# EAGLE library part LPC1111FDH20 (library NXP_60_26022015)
32-bit ARM Cortex-M0 microcontroller; up to 64 kB flash and 8 kB SRAM The LPC1110/11/12/13/14/15 are a ARM Cortex-M0 based, low-cost 32-bit MCU family, designed for 8/16-bit microcontroller applications, offering performance, low power, simple instruction set and memory addressing together with reduced code size compared to existing 8/16-bit architectures. The LPC1110/11/12/13/14/15 operate at CPU frequencies of up to 50 MHz. The peripheral complement of the LPC1110/11/12/13/14/15 includes up to 64 kB of flash memory, up to 8 kB of data memory, one Fast-mode Plus I 2 C-bus interface, one RS-485/EIA-485 UART, up to two SPI interfaces with SSP features, four general purpose counter/timers, a 10-bit ADC, and up to 42 general purpose I/O pins. Remark: The LPC111x series consists of the LPC1100 series (parts LPC111x/101/201/301), LPC1100L series (parts LPC111x/002/102/202/302), and the LPC1100XL series (parts LPC111x/103/203/303/323/333). The LPC1100L and LPC1100XL series include the power profiles, a windowed watchdog timer, and a configurable open-drain mode. AAL Eindhoven MK
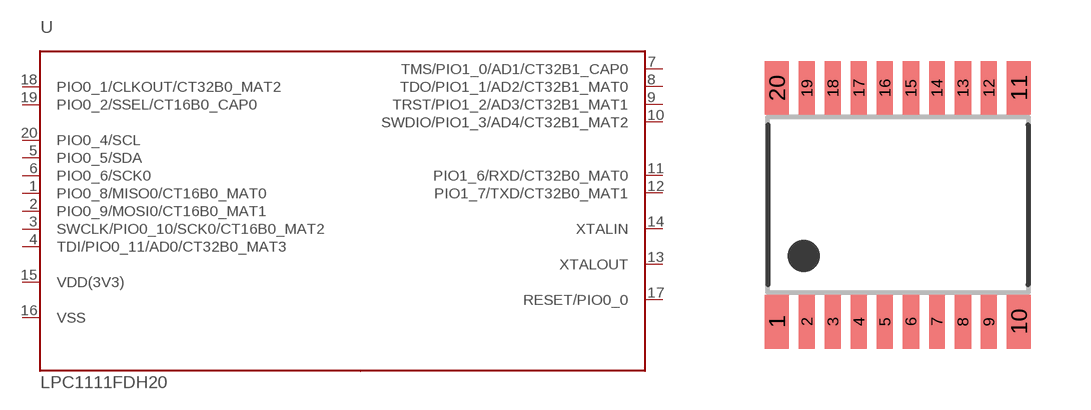
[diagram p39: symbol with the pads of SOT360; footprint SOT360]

Designator prefix U

## LPC1111FDH20/002 (ADC: 5; FLASH: 8kB; GPIO: 16; PWR_PROFILES: yes; SERIES: LPC1100L; SPI: 1; SRAM: 2kB)  [SOT360]
1  PIO0_8/MISO0/CT16B0_MAT0
2  PIO0_9/MOSI0/CT16B0_MAT1
3  SWCLK/PIO0_10/SCK0/CT16B0_MAT2
4  TDI/PIO0_11/AD0/CT32B0_MAT3
5  PIO0_5/SDA
6  PIO0_6/SCK0
7  TMS/PIO1_0/AD1/CT32B1_CAP0
8  TDO/PIO1_1/AD2/CT32B1_MAT0
9  TRST/PIO1_2/AD3/CT32B1_MAT1
10  SWDIO/PIO1_3/AD4/CT32B1_MAT2
11  PIO1_6/RXD/CT32B0_MAT0
12  PIO1_7/TXD/CT32B0_MAT1
13  XTALOUT  out
14  XTALIN  in
15  VDD(3V3)  pwr
16  VSS  pwr
17  RESET/PIO0_0
18  PIO0_1/CLKOUT/CT32B0_MAT2
19  PIO0_2/SSEL/CT16B0_CAP0
20  PIO0_4/SCL

## Footprint SOT360 (pad centres in mm)
SOT360 TSSOP20: plastic thin shrink small outline package; 20 leads; body width 4.4 mm JEDEC: MO-153 IEC:
smd 0.6 x 1.35: 1 -3.025,-2.925; 10 3.025,-2.925; 11 3.025,2.925; 20 -3.025,2.925
smd 0.4 x 1.35: 2 -2.275,-2.925; 3 -1.625,-2.925; 4 -0.975,-2.925; 5 -0.325,-2.925; 6 0.325,-2.925; 7 0.975,-2.925; 8 1.625,-2.925; 9 2.275,-2.925; 12 2.275,2.925; 13 1.625,2.925; 14 0.975,2.925; 15 0.325,2.925; 16 -0.325,2.925; 17 -0.975,2.925; 18 -1.625,2.925; 19 -2.275,2.925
